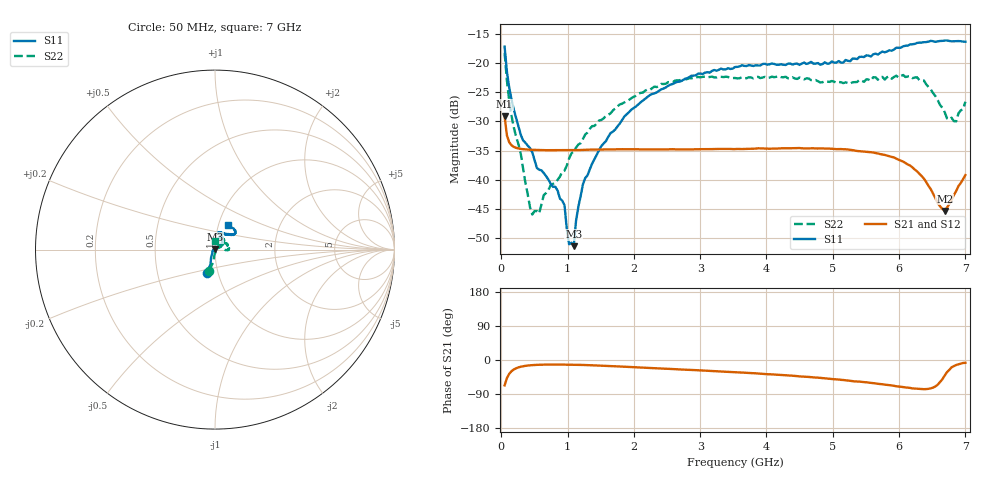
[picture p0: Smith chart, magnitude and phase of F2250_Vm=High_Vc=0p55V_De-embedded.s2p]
! Integrated Device Technology
! Corporate Headquarters
! 6024 Silver Creek Valley Road
! San Jose, CA 95138  USA
! Phone:  1-408-284-8200
! Toll Free:  1-800-223-1366
! Webpage:  http://www.idt.com/
! Timing and RF Division
! 515 Groton Road, Suite 102
! Westford, MA 01886-6024
! Device:  F2250
! Description: Voltage Variable RF Attenuator
! Frequency:  50.0 -  6000.00 MHz
! Package:  3x3 mm Thin QFN Plastic Package: 16 pin
! Ports:  2 RF, 3 DC
!  Pin  1  = GND
!  Pin  2  = NC
!  Pin  3  = RF1  = Port 1
!  Pin  4  = NC
!  Pin  5  = GND
!  Pin  6  = GND
!  Pin  7  = GND
!  Pin  8  = GND
!  Pin  9  = NC
!  Pin 10  = RF2  = Port 2
!  Pin 11  = NC
!  Pin 12  = GND
!  Pin 13  = GND
!  Pin 14  = VCNTRL
!  Pin 15  = VDD
!  Pin 16  = VMODE
! Vcntrl:  0.550 Volts
! Vmode:  +3.300 Volts
! Vdd:  +3.30  Volts
! Current:  1.272 mA
! Data:  The device was measured on a the F2250 evaluation board which has
!  individual transmission lines to the RF pins.  Data was collected
!  using a calibrated network analyzer.  The evaluation board was
!  de-embedded using a TRL calibration technique.
!  The reference plane is the edge of the package pin.
! Misc:  SN 10
!  Action Tracker AT0258
! Date Measured:  2014-11-26
! Date:  2015-10-15  MJV
! Note:
!  Integrated Device Technology supplies this data as a sample of measured
!  data at the package pin for this product.  Your particular data for this
!  product may vary.
!  Data was taken at 25 degrees C.
!  Integrated Device Technology reserves the right to change this data at anytime.
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# GHz S dB R 50
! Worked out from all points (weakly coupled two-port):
!   201 points, 50 MHz to 7 GHz, reference 50 ohm
!   highest |S21| = -29.14 dB at 50 MHz (marker M1); lowest = -45.4 dB at 6.687 GHz (marker M2)
!   lowest |S11| = -51.4 dB at 1.093 GHz (marker M3), VSWR 1.01, Z = 50 + j0.268 ohm
!   |S11| at or under -10 dB: start of sweep to end of sweep
!   |S22| runs from -46.0 to -18.2 dB; largest |S21 - S12| = 6.4e-05
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0.05  -17.17 -108.4  -29.14 -66.9  -29.14 -66.9  -18.21 -106.1
0.08475  -21.47 -107.3  -32.41 -47.8  -32.42 -47.8  -22.99 -97.9
0.189  -28.01 -119.8  -34.38 -25.0  -34.38 -25.0  -31.04 -95.0
0.328  -33.25 -133.7  -34.77 -16.5  -34.77 -16.5  -38.07 -75.4
0.467  -35.30 -145.8  -34.88 -13.5  -34.88 -13.5  -45.99 -47.4
0.57125  -38.31 -160.8  -34.92 -12.6  -34.92 -12.6  -45.79 -12.7
0.64075  -38.87 -162.2  -34.94 -12.2  -34.94 -12.2  -42.66 7.6
0.9535  -44.39 171.1  -34.96 -12.1  -34.96 -12.1  -38.46 29.4
1.023  -51.10 139.7  -34.95 -12.3  -34.96 -12.3  -36.36 28.5
1.0925  -51.43 87.1  -34.94 -12.5  -34.94 -12.5  -35.15 29.6
1.12725  -47.09 59.7  -34.93 -12.6  -34.93 -12.6  -34.51 26.9
1.2315  -40.79 40.0  -34.90 -13.1  -34.90 -13.1  -33.02 23.8
1.6485  -32.01 40.9  -34.82 -16.0  -34.83 -16.0  -28.61 31.0
2.37825  -24.75 46.5  -34.80 -22.2  -34.81 -22.2  -23.93 37.6
3.525  -20.66 71.6  -34.76 -32.2  -34.75 -32.3  -22.55 63.5
4.7065  -20.07 71.9  -34.63 -45.8  -34.63 -45.8  -22.94 64.5
5.2625  -19.67 53.2  -34.87 -55.0  -34.87 -55.0  -23.53 43.1
5.85325  -17.80 40.5  -35.99 -66.4  -35.99 -66.6  -22.26 14.4
6.3745  -16.41 40.9  -39.83 -77.0  -39.84 -77.0  -22.98 -2.1
6.68725  -16.12 47.8  -45.36 -41.2  -45.36 -41.0  -28.41 19.9
6.861  -16.22 54.5  -41.96 -13.2  -41.93 -13.1  -29.99 59.3
7  -16.33 62.4  -39.21 -7.5  -39.17 -7.7  -26.62 91.6
